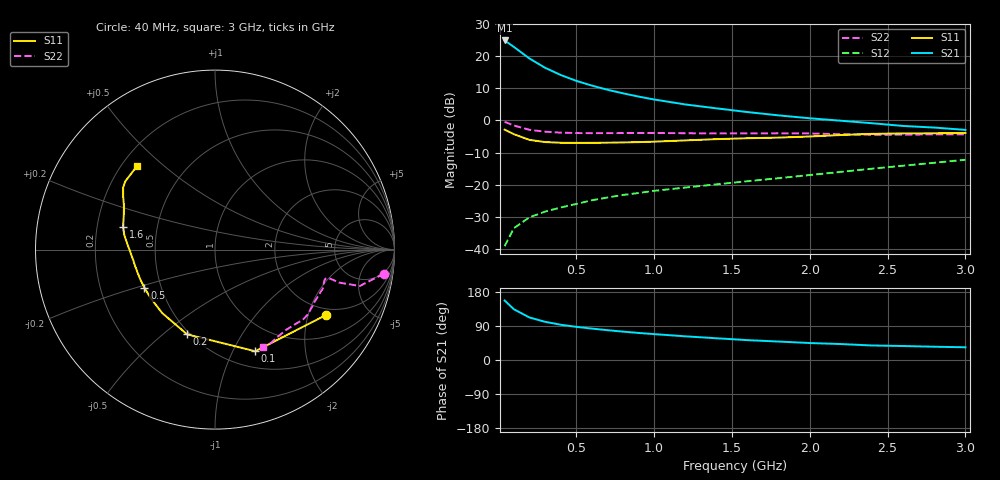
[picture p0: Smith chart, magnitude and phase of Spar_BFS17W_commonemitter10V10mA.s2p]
! Filename:  BFS17WH.S2P  Version:  4.0
! NXP part #: BFS17W  Date: Jun 1994
! Bias condition: Vce=10V, Ic=10mA
#  MHz  S  MA  R  50
! Freq  S11  S21  S12  S22  !GUM [dB]
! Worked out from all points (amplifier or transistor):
!   21 points, 40 MHz to 3 GHz, reference 50 ohm
!   highest |S21| = 24.9 dB at 40 MHz (marker M1)
!   |S21| within 3 dB of that: start of sweep to 126.9 MHz
!   unconditionally stable (mu >= 1): 436.7 MHz to 2.408 GHz
!   at 300 MHz: K = 0.84, MSG = 22.4 dB, |S12| = -28.4 dB
!   at 1 GHz: K = 1.19, MAG = 11.6 dB, |S12| = -21.9 dB
!   at 3 GHz: K = 0.94, MSG = 4.7 dB, |S12| = -12.3 dB
!   S11 on the Smith chart (normalised r, x): 40 MHz: 1.74, -2.62; 100 MHz: 0.68, -1.23; 200 MHz: 0.48, -0.61; 500 MHz: 0.40, -0.21; 1.6 GHz: 0.31, +0.11; 3 GHz: 0.26, +0.41
40  0.718 -30.5  17.6 157.1  0.011 74.3  0.951 -8.1
100  0.609 -68.4  13.93 133.7  0.021 61.6  0.832 -14.1
200  0.497 -108.2  9.202 112.1  0.031 55.9  0.714 -14.9
300  0.46 -129.7  6.605 100.8  0.038 56.5  0.667 -14.2
400  0.449 -142.9  5.102 93.1  0.044 58.5  0.645 -14.2
500  0.447 -151.5  4.137 87.5  0.05 60.8  0.636 -14.8
600  0.448 -158.1  3.489 82.9  0.057 63.0  0.633 -15.8
700  0.45 -163.4  3.005 78.7  0.063 64.4  0.634 -16.8
800  0.454 -168.1  2.644 74.9  0.069 66.0  0.636 -17.9
900  0.459 -172.4  2.353 71.4  0.074 67.2  0.638 -18.9
1000  0.467 -176.3  2.119 68.3  0.08 68.8  0.638 -20.1
1200  0.488 176.7  1.774 62.5  0.09 71.5  0.632 -23.0
1400  0.511 171.1  1.543 57.4  0.101 74.6  0.627 -26.8
1600  0.528 166.0  1.35 52.4  0.113 77.5  0.628 -31.3
1800  0.54 160.4  1.198 48.7  0.126 80.9  0.631 -35.0
2000  0.562 154.5  1.08 44.8  0.141 83.7  0.626 -38.6
2200  0.592 149.8  0.989 42.1  0.158 86.1  0.61 -43.0
2400  0.618 145.9  0.904 38.3  0.177 87.8  0.597 -48.9
2600  0.628 142.8  0.82 36.9  0.197 88.8  0.599 -54.9
2800  0.63 138.1  0.774 35.0  0.219 89.7  0.608 -59.8
3000  0.637 132.7  0.712 33.6  0.244 90.1  0.607 -63.6
